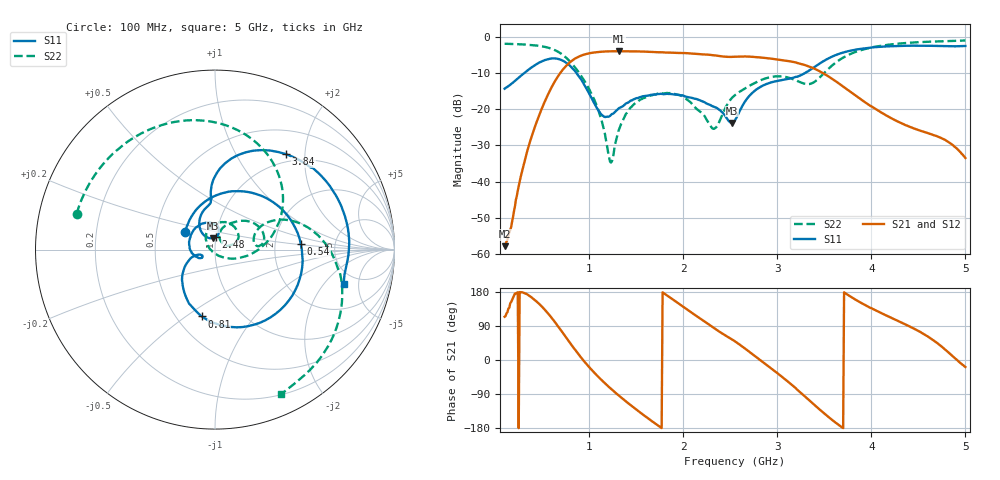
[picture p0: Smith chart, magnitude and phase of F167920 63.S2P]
!  2-Port S-parameters saved by WinCal
! VAR MeasName=S-Parameters (CALIBRATED_DATA) read from VNA (N5242A)
! VAR MeasDate=2016-11-22 9:58:40
! VAR NAME=F167920 63
! VAR FILENAME=F167920 63.S2P
! VAR DATE=2016-11-22 9:58:40
! VAR PHYS_PORTS=1,2
# Hz S DB R 50
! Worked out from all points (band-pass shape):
!   491 points, 100 MHz to 5 GHz, reference 50 ohm
!   highest |S21| = -4.02 dB at 1.32 GHz (marker M1); lowest = -57.8 dB at 100 MHz (marker M2)
!   |S21| within 3 dB of the highest: 797.6 MHz to 3.177 GHz (2.379 GHz wide, 120 % of centre)
!   lowest |S11| = -23.8 dB at 2.52 GHz (marker M3), VSWR 1.14, Z = 48.3 + j6.13 ohm
!   |S11| at or under -10 dB: start of sweep to 310.4 MHz; 862.5 MHz to 3.298 GHz (2.435 GHz wide, 117 % of centre)
!   |S22| runs from -34.7 to -1.1 dB; largest |S21 - S12| = 0.0011
!   S11 on the Smith chart (normalised r, x): 100 MHz: 0.70, +0.14; 540 MHz: 2.82, +0.22; 810 MHz: 0.66, -0.58; 2.48 GHz: 1.00, +0.14; 3.84 GHz: 0.87, +1.64; 5 GHz: 3.83, -3.28
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1e8  -14.36 149.8  -57.75 114.1  -57.09 108.5  -1.98 165.5
3.6e8  -9.00 66.6  -29.81 169.8  -29.82 169.7  -2.27 125.7
5.4e8  -6.39 3.6  -17.15 129.1  -17.16 129.2  -2.91 92.6
6.9e8  -6.31 -54.6  -10.10 81.7  -10.09 81.7  -4.53 58.7
8.1e8  -8.41 -101.3  -6.76 40.0  -6.75 40.0  -7.28 30.2
9.2e8  -12.05 -137.4  -5.17 4.4  -5.16 4.4  -11.09 6.3
1.1e9  -20.47 -162.9  -4.25 -45.3  -4.24 -45.3  -20.50 -31.7
1.23e9  -21.63 -148.3  -4.07 -75.7  -4.07 -75.7  -34.72 -132.9
1.32e9  -19.66 -154.2  -4.02 -95.0  -4.02 -95.0  -25.38 143.7
1.48e9  -17.19 -179.2  -4.09 -126.7  -4.09 -126.7  -18.54 108.7
1.74e9  -15.84 135.2  -4.31 -174.4  -4.31 -174.4  -15.68 67.1
2.06e9  -16.75 94.5  -4.62 129.9  -4.62 129.9  -17.77 20.4
2.32e9  -19.28 78.9  -5.12 85.4  -5.13 85.4  -25.43 39.8
2.48e9  -23.17 85.9  -5.59 60.1  -5.59 60.1  -18.17 71.6
2.52e9  -23.79 102.1  -5.59 54.0  -5.59 54.0  -16.83 66.9
2.55e9  -23.08 115.0  -5.55 49.2  -5.55 49.2  -16.12 63.5
2.9e9  -12.92 106.4  -5.98 -15.4  -5.99 -15.5  -11.33 29.8
3.15e9  -11.47 94.9  -6.88 -64.7  -6.90 -64.8  -11.57 6.5
3.37e9  -8.81 92.8  -8.57 -113.1  -8.58 -113.1  -12.84 18.0
3.84e9  -3.57 53.3  -16.42 157.9  -16.44 157.9  -4.16 2.5
4.19e9  -2.67 26.3  -22.20 113.9  -22.21 114.1  -2.21 -24.8
5e9  -2.59 -15.0  -33.46 -18.5  -33.45 -18.8  -1.07 -65.2
